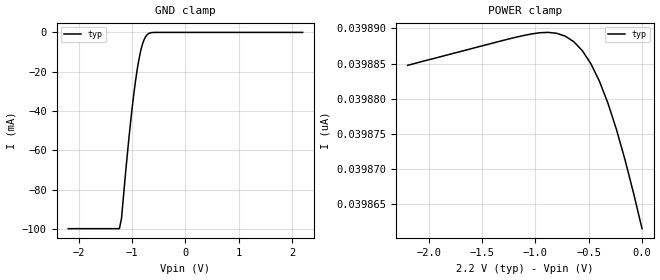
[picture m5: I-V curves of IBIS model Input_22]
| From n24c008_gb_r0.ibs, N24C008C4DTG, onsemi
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|//////////////////////////////////////////////////////////////////////////////
|//////////////////////////////////////////////////////////////////////////////
[Model]  Input_22
Model_type Input
Vinh =  0.96
Vinl =  0.24
|  variable   typ   min   max
C_comp   3.8pF   3.8pF   3.8pF
|//////////////////////////////////////////////////////////////////////////////
[Temperature Range]   25   125   -40
|//////////////////////////////////////////////////////////////////////////////
[Voltage Range]   2.20V   2.20V   2.20V
|//////////////////////////////////////////////////////////////////////////////
[POWER Clamp Reference] 2.20V   2.20V   2.20V
|//////////////////////////////////////////////////////////////////////////////
[GND Clamp Reference]   0V   0V   0V
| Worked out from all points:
|   GND clamp passes 1 mA (typ) near -0.71 V on its own axis
|//////////////////////////////////////////////////////////////////////////////
[GND Clamp]
|   Voltage   I(typ)   I(min)   I(max)
-2.2V     -99.88mA   NA         NA
-1.24V    -99.88mA   NA         NA
-1.2V     -94.64mA   NA         NA
-1.12V    -70.4mA    NA         NA
-1.04V    -48.28mA   NA         NA
-980mV    -33.74mA   NA         NA
-920mV    -21.46mA   NA         NA
-880mV    -14.81mA   NA         NA
-820mV    -7.235mA   NA         NA
-760mV    -2.799mA   NA         NA
-700mV    -756uA     NA         NA
2.2V      39.86nA    NA         NA
|//////////////////////////////////////////////////////////////////////////////
[POWER Clamp]
|   Voltage   I(typ)   I(min)   I(max)
-2.2V     39.88nA    NA         NA
-1.2V     39.89nA    NA         NA
-960mV    39.89nA    NA         NA
-800mV    39.89nA    NA         NA
-640mV    39.89nA    NA         NA
-560mV    39.89nA    NA         NA
-480mV    39.88nA    NA         NA
-400mV    39.88nA    NA         NA
-320mV    39.88nA    NA         NA
-240mV    39.88nA    NA         NA
-160mV    39.87nA    NA         NA
0V        39.86nA    NA         NA
